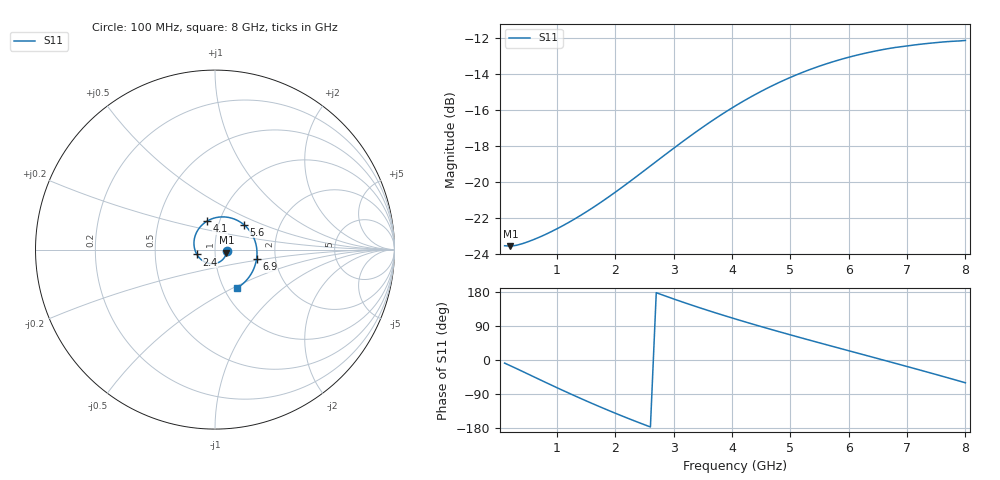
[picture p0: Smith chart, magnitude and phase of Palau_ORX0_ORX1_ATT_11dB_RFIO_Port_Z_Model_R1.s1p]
! Created Fri Oct  9 14:28:12 2020
! Palau ORX0/ORX1 RFIO Port Impedance Model.
! Attenuation  : 11 dB.
! Revision		: R1.
! Impedance Mode 	: Balanced Differential-Mode.
! Impedance Format 	: Series Equivalent Differential Impedance (SEDZ).
# hz S ma R 100
! 1 Port Network Data from SP1.SP block
! freq  magS11  angS11
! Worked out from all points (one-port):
!   80 points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, 100 MHz to 8 GHz, reference 100 ohm
!   lowest |S11| = -23.6 dB at 200 MHz (marker M1), VSWR 1.14, Z = 114 - j3.97 ohm
!   |S11| at or under -10 dB: start of sweep to end of sweep
!   S11 on the Smith chart (normalised r, x): 100 MHz: 1.14, -0.02; 2.4 GHz: 0.82, -0.04; 4.1 GHz: 0.87, +0.28; 5.6 GHz: 1.32, +0.38; 6.9 GHz: 1.59, -0.18; 8 GHz: 1.15, -0.53
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1e8  0.06637 -8.2
2e8  0.06619 -15.2
6e8  0.06906 -44.3
1.1e9  0.07549 -80.3
1.4e9  0.08054 -101.2
1.6e9  0.08444 -114.6
1.8e9  0.08878 -127.8
2.1e9  0.09615 -146.8
2.4e9  0.1045 -165.1
2.8e9  0.1171 172.0
3.1e9  0.1274 155.7
3.3e9  0.1346 145.2
3.6e9  0.1456 130.1
4.1e9  0.1641 106.3
4.4e9  0.1749 92.6
4.6e9  0.1819 83.7
4.9e9  0.1919 70.7
5.1e9  0.1982 62.1
5.3e9  0.2041 53.6
5.6e9  0.2123 41.0
6.1e9  0.2241 20.3
6.5e9  0.2316 3.7
6.7e9  0.2349 -4.6
6.9e9  0.2374 -13.0
7.1e9  0.2398 -21.4
7.5e9  0.2437 -38.4
7.7e9  0.2453 -47.0
8e9  0.2471 -60.1
